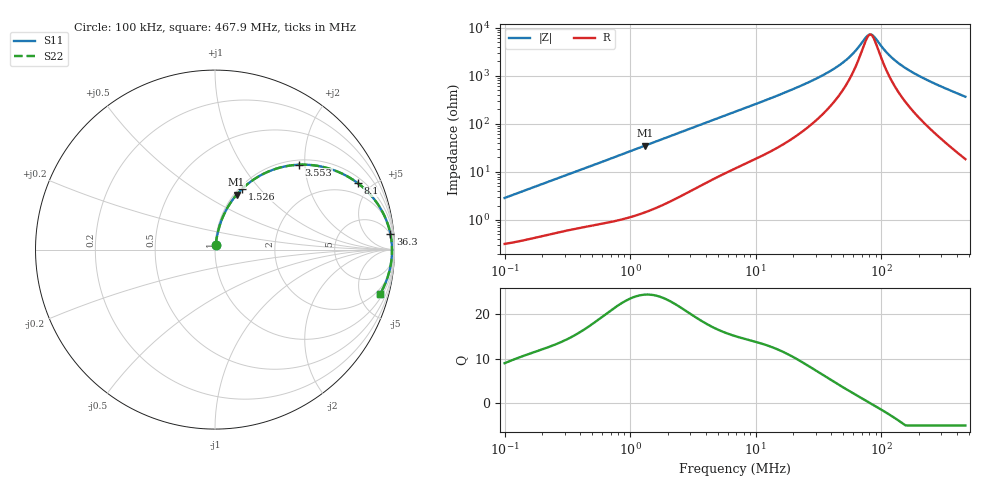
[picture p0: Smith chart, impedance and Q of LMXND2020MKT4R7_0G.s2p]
! LMXND2020MKT4R7_0G  S-PARAMETER MODEL  ( General Type )
! Model Generated by TAIYO YUDEN Corporation (https://www.yuden.co.jp/en/)
! Version 1.0
! TAIYO YUDEN Control No. 191023NI43SB-FBB
! Copyright(c) 2019 TAIYO YUDEN CO.,LTD. All Rights Reserved.
! Product Description (link to TY-COMPAS)
! https://ds.yuden.co.jp/TYCOMPAS/or/detail?pn=LMXND2020MKT4R7M0G&u=M
! Products Name : Inductors
! Characteristics :
!  Inductance : 4.7 uH , SRF(min) : -Hz , DC Resistance(max) : 0.2892 Ohm
!  Rated Current : Saturation :900 mA , Temp Rise : 910 mA (40 degC)
!  Case Size : 2.0 x 2.0 / 0.079 x 0.079 [mm/inch] , Thickness : 1.2 / 0.047 [mm/inch]
!  (Conditions: Temperature = 25 degC , DC Bias Current/Voltage = 0A / 0V)
! External Node Assignments :
!  1  o---GGG---o  2
! GND o---------o GND
! Frequency Range : 0.1MHz  -  467.920999MHz  [ 402 STEP ]
# MHz S RI R 50
! Freq[MHz].  S11 Real  S11 Imag  S21 Real  S21 Imag  S12 Real  S12 Imag  S22 Real  S22 Imag
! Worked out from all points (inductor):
!   401 points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, 100 kHz to 467.9 MHz, reference 50 ohm
!   read as one part in series: L = 4.52 uH near 104.3 kHz
!   highest Q = 24.3 at 1.316 MHz (marker M1), where L = 4.25 uH
!   self-resonance near 81.02 MHz
!   S11 on the Smith chart (normalised r, x): 100 kHz: 1.01, +0.06; 1.526 MHz: 1.03, +0.81; 3.553 MHz: 1.10, +1.87; 8.1 MHz: 1.29, +4.16; 36.3 MHz: 5, +22; 467.9 MHz: 1.37, -7.29
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0.1  0.00398 0.0283  0.996 -0.0283  0.996 -0.0283  0.00398 0.0283
0.411864  0.0191 0.1095  0.9809 -0.1095  0.9809 -0.1095  0.0191 0.1095
0.809781  0.0538 0.204  0.9462 -0.204  0.9462 -0.204  0.0538 0.204
1.316445  0.12 0.3051  0.88 -0.3051  0.88 -0.3051  0.12 0.3051
1.526267  0.1524 0.3394  0.8476 -0.3394  0.8476 -0.3394  0.1524 0.3394
1.69632  0.1799 0.3638  0.8201 -0.3638  0.8201 -0.3638  0.1799 0.3638
2.534201  0.3187 0.4432  0.6813 -0.4432  0.6813 -0.4432  0.3187 0.4432
3.553431  0.4681 0.473  0.5319 -0.473  0.5319 -0.473  0.4681 0.473
6.986533  0.7507 0.4005  0.2493 -0.4005  0.2493 -0.4005  0.7507 0.4005
8.100088  0.7969 0.3692  0.2031 -0.3692  0.2031 -0.3692  0.7969 0.3692
14.02978  0.9121 0.2456  0.0879 -0.2456  0.0879 -0.2456  0.9121 0.2456
28.17346  0.9694 0.1199  0.0306 -0.1199  0.0306 -0.1199  0.9694 0.1199
36.30324  0.9776 0.0857  0.0224 -0.0857  0.0224 -0.0857  0.9776 0.0857
54.23486  0.9843 0.0404  0.0157 -0.0404  0.0157 -0.0404  0.9843 0.0404
62.87913  0.9854 0.0254  0.0146 -0.0254  0.0146 -0.0254  0.9854 0.0254
76.04759  0.9862 0.00695  0.0138 -0.00695  0.0138 -0.00695  0.9862 0.00695
81.02364  0.9863 0.00087  0.0137 -0.00087  0.0137 -0.00087  0.9863 0.00087
88.1685  0.9863 -0.00724  0.0137 0.00724  0.0137 0.00724  0.9863 -0.00724
116.0364  0.9852 -0.0342  0.0148 0.0342  0.0148 0.0342  0.9852 -0.0342
146.3942  0.9829 -0.0589  0.0171 0.0589  0.0171 0.0589  0.9829 -0.0589
196.7795  0.9773 -0.0947  0.0227 0.0947  0.0227 0.0947  0.9773 -0.0947
467.921  0.9194 -0.2481  0.0806 0.2481  0.0806 0.2481  0.9194 -0.2481
